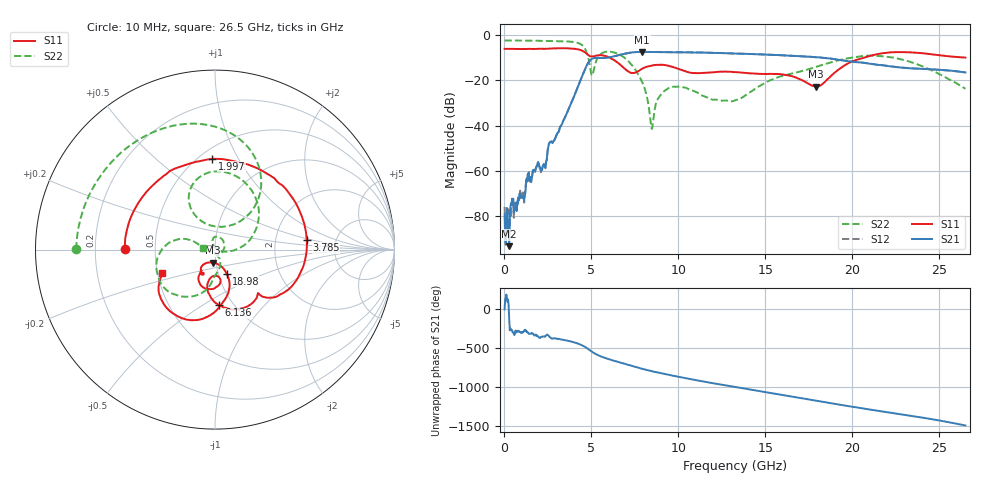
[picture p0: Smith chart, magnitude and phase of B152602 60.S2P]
!  2-Port S-parameters saved by WinCal
! VAR MeasName=S-Parameters (CALIBRATED_DATA) read from VNA (N5242A)
! VAR MeasDate=2016-1-5 16:34:23
! VAR NAME=B152602 60
! VAR FILENAME=B152602 60.S2P
! VAR DATE=2016-1-5 16:34:23
! VAR PHYS_PORTS=1,2
# Hz S DB R 50
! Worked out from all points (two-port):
!   801 points, 10 MHz to 26.5 GHz, reference 50 ohm
!   highest |S21| = -7.31 dB at 7.924 GHz (marker M1); lowest = -93.5 dB at 274.9 MHz (marker M2)
!   |S21| within 3 dB of the highest: 5.055 GHz to 18.78 GHz (13.72 GHz wide, 115 % of centre)
!   lowest |S11| = -22.7 dB at 17.92 GHz (marker M3), VSWR 1.16, Z = 48.3 - j7.03 ohm
!   |S11| at or under -10 dB: 6.087 GHz to 20.62 GHz (14.54 GHz wide, 109 % of centre)
!   |S22| runs from -41.5 to -2.2 dB; largest |S21 - S12| = 0.003
!   S11 on the Smith chart (normalised r, x): 10 MHz: 0.33, +0.00; 1.997 GHz: 0.58, +0.79; 3.785 GHz: 3.04, +0.44; 6.136 GHz: 0.86, -0.59; 18.98 GHz: 1.10, -0.30; 26.5 GHz: 0.53, -0.15
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1e7  -5.96 179.6  -79.12 1.7  -76.10 77.8  -2.25 179.8
2.749e8  -5.97 167.8  -93.51 -126.2  -86.02 -169.4  -2.25 175.8
1.99675e9  -5.91 91.7  -57.66 -2.2  -57.92 -4.5  -2.39 148.3
2.294762e9  -5.96 77.8  -57.22 11.9  -57.43 9.5  -2.43 143.0
2.625888e9  -5.84 62.8  -47.31 1.6  -47.39 1.5  -2.45 136.7
3.784825e9  -5.78 6.0  -31.00 -50.4  -31.00 -50.2  -2.78 107.5
4.447075e9  -6.73 -29.8  -18.47 -99.5  -18.45 -99.3  -4.19 75.1
5.0431e9  -9.37 -45.3  -10.36 174.5  -10.34 174.6  -17.82 87.7
6.135812e9  -10.18 -85.9  -9.56 70.9  -9.55 71.1  -7.29 78.3
7.129188e9  -16.06 -98.4  -7.80 5.4  -7.78 5.3  -11.49 28.7
7.923888e9  -14.75 -80.6  -7.31 -44.4  -7.32 -44.3  -20.80 -5.1
8.453688e9  -13.43 -89.7  -7.36 -72.9  -7.36 -72.9  -41.21 36.2
8.851038e9  -13.05 -98.8  -7.42 -93.0  -7.39 -93.1  -27.78 108.5
9.579512e9  -13.81 -115.3  -7.47 -127.0  -7.47 -127.1  -22.90 89.0
1.083779e10  -16.68 -118.5  -7.51 178.1  -7.50 178.1  -24.53 28.8
1.3255e10  -16.29 -121.2  -8.05 81.7  -8.03 81.6  -28.80 -70.5
1.53742e10  -17.10 -122.8  -8.61 1.7  -8.58 1.8  -19.65 -75.6
1.769208e10  -22.27 -112.1  -9.53 -85.6  -9.52 -85.4  -14.55 -96.0
1.792386e10  -22.71 -99.2  -9.68 -94.3  -9.65 -94.4  -13.97 -97.9
1.898346e10  -16.53 -63.9  -10.56 -135.3  -10.52 -135.0  -11.49 -110.0
2.209604e10  -7.57 -110.4  -13.67 114.8  -13.59 114.6  -9.56 -167.8
2.65e10  -9.83 -156.6  -16.44 -52.5  -16.44 -52.7  -23.69 173.7
